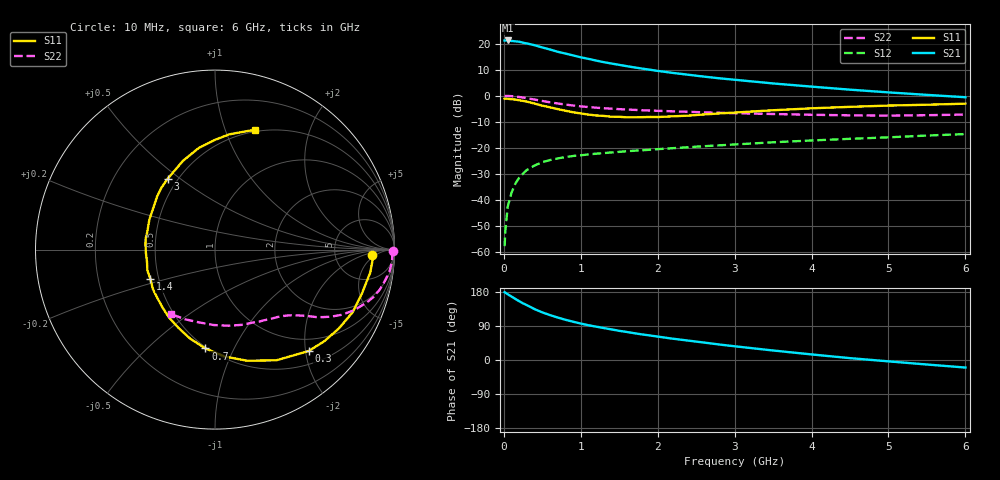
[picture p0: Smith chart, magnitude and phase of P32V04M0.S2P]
! SIEMENS Small Signal Semiconductors
! BFP181
! Si NPN RF Bipolar Junction Transistor in SOT143
! VCE = 2 V  IC = 4 mA
! Common Emitter S-Parameters:  March  1996
# GHz  S  MA  R  50
!  f  S11  S21  S12  S22
! GHz  MAG  ANG  MAG  ANG  MAG  ANG  MAG  ANG
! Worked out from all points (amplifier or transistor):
!   36 points, 10 MHz to 6 GHz, reference 50 ohm
!   highest |S21| = 21.2 dB at 50 MHz (marker M1)
!   |S21| within 3 dB of that: start of sweep to 539.9 MHz
!   unconditionally stable (mu >= 1): 1.782 GHz to end of sweep
!   at 250 MHz: K = 0.20, MSG = 25.1 dB, |S12| = -29.9 dB
!   at 1.4 GHz: K = 0.87, MSG = 17.0 dB, |S12| = -21.8 dB
!   at 6 GHz: K = 1.07, MAG = 5.5 dB, |S12| = -14.7 dB
!   S11 on the Smith chart (normalised r, x): 10 MHz: 14, -3; 300 MHz: 0.75, -2.06; 700 MHz: 0.49, -0.78; 1.4 GHz: 0.45, -0.17; 3 GHz: 0.44, +0.45; 6 GHz: 0.48, +1.27
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0.01  0.8727 -1.8  11.46 178.8  0.0013 80.7  0.9918 -0.6
0.02  0.8803 -3.6  11.45 177.8  0.0026 83.4  0.9877 -1.4
0.05  0.8743 -8.4  11.47 173.5  0.0074 89.3  0.9888 -3.6
0.15  0.8427 -24.5  11.05 161.1  0.0206 76.3  0.9627 -10.4
0.2  0.818 -32.5  10.84 155.1  0.0267 72.1  0.9443 -13.7
0.25  0.7946 -40.0  10.38 149.4  0.032 68.1  0.9208 -16.7
0.3  0.769 -47.3  10.05 144.7  0.0377 64.8  0.8959 -19.2
0.4  0.7052 -61.0  9.289 134.2  0.0459 59.0  0.8437 -23.7
0.5  0.6445 -73.9  8.422 125.6  0.053 53.1  0.7923 -27.3
0.6  0.5983 -84.8  7.692 118.5  0.0583 49.5  0.7472 -30.0
0.7  0.5535 -95.5  6.965 112.1  0.0626 46.4  0.7097 -32.0
0.8  0.5154 -105.5  6.436 106.2  0.0664 43.7  0.6774 -33.7
0.9  0.4815 -115.0  5.93 101.0  0.0698 41.8  0.6486 -35.0
1.1  0.4343 -132.7  5.09 91.7  0.0748 39.1  0.6053 -37.4
1.4  0.3951 -155.7  4.14 80.7  0.0817 36.6  0.5636 -40.5
1.8  0.3878 176.4  3.308 67.4  0.0897 34.9  0.5259 -44.7
2.2  0.4025 155.2  2.734 56.1  0.0986 33.3  0.5016 -49.6
3  0.475 123.6  2.023 36.2  0.116 30.2  0.4612 -61.3
3.5  0.5261 109.8  1.719 25.1  0.1278 28.1  0.4455 -70.2
4.5  0.6114 90.0  1.306 4.9  0.1489 22.7  0.4203 -91.0
5.5  0.6716 77.2  1.037 -11.9  0.1721 17.6  0.4227 -113.4
6  0.7034 71.6  0.935 -19.9  0.1839 14.2  0.4352 -124.7
